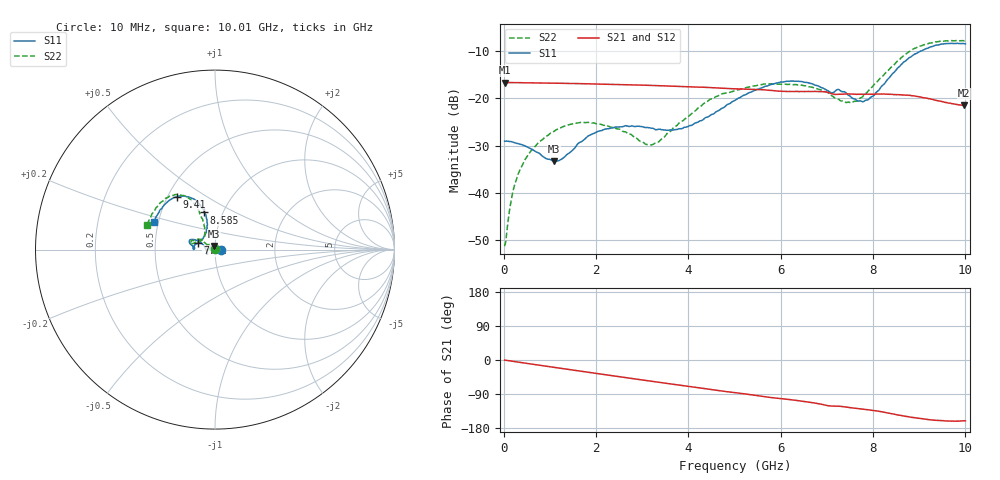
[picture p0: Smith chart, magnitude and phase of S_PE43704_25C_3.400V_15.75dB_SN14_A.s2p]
! Device ID: PE43704
! Dir: z:\PE43704\PE43704_Char_1_20130516\PE43704\AMB\3p400V\15p75dB
! Serial: 14
! Insertion: A
! Impedance: 50 ohm
! Temp: Amb
! VDD: 3.400V
! Attenuation Step: 15.75dB
! IDD: 1.139951e-01mA
#  Hz  S  RI  R  50
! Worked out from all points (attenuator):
!   401 points, 10 MHz to 10.01 GHz, reference 50 ohm
!   highest |S21| = -16.73 dB at 10 MHz (marker M1); lowest = -21.6 dB at 9.985 GHz (marker M2)
!   lowest |S11| = -33.3 dB at 1.085 GHz (marker M3), VSWR 1.04, Z = 49.4 + j2.07 ohm
!   |S11| at or under -10 dB: start of sweep to 9.074 GHz
!   |S22| runs from -51.2 to -7.9 dB; largest |S21 - S12| = 0.0013
!   S11 on the Smith chart (normalised r, x): 10 MHz: 1.07, +0.00; 7.51 GHz: 0.82, +0.06; 8.585 GHz: 0.82, +0.36; 9.41 GHz: 0.56, +0.38; 10.01 GHz: 0.47, +0.17
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1e7  0.0351 0.000273  0.1458 -0.000522  0.1459 -0.00048  -0.00269 0.000566
1.85e8  0.0336 0.00728  0.1452 -0.0087  0.1451 -0.00871  -0.00289 0.00969
3.6e8  0.0297 0.0133  0.1442 -0.0167  0.1441 -0.0169  -0.00614 0.0171
6.35e8  0.0192 0.0208  0.1416 -0.0288  0.1415 -0.0287  -0.0147 0.0258
1.085e9  -0.0054 0.0209  0.1353 -0.0477  0.1354 -0.0476  -0.0348 0.028
1.685e9  -0.0347 0.00293  0.1229 -0.0708  0.1229 -0.0706  -0.0543 0.0121
2.41e9  -0.045 -0.0203  0.1027 -0.0941  0.1027 -0.0941  -0.048 -0.00319
3.11e9  -0.0424 -0.0244  0.079 -0.1111  0.0791 -0.111  -0.0318 0.006
3.36e9  -0.0426 -0.0198  0.0697 -0.1156  0.0698 -0.1155  -0.0319 0.0139
4.035e9  -0.0513 0.00382  0.0443 -0.1235  0.0444 -0.1233  -0.0549 0.0369
4.46e9  -0.0614 0.0212  0.0282 -0.1261  0.0283 -0.1262  -0.0788 0.0555
5.01e9  -0.0848 0.0418  0.0083 -0.1246  0.0084 -0.1248  -0.1071 0.0529
5.96e9  -0.1344 0.0561  -0.023 -0.1161  -0.023 -0.1161  -0.134 0.0406
6.685e9  -0.138 0.0314  -0.0449 -0.1081  -0.0451 -0.1082  -0.1255 0.0334
7.51e9  -0.0973 0.0378  -0.0644 -0.0895  -0.0642 -0.0895  -0.0677 0.0584
7.86e9  -0.0626 0.0716  -0.0718 -0.0831  -0.0715 -0.0833  -0.0567 0.0974
8.36e9  -0.0446 0.1579  -0.0846 -0.0697  -0.0844 -0.07  -0.0763 0.1861
8.585e9  -0.0599 0.2071  -0.0894 -0.061  -0.0887 -0.0614  -0.101 0.234
8.935e9  -0.106 0.2733  -0.093 -0.0476  -0.093 -0.0468  -0.1626 0.2949
9.41e9  -0.2125 0.2925  -0.088 -0.0328  -0.0881 -0.0324  -0.2628 0.2905
9.985e9  -0.3336 0.1661  -0.0788 -0.0281  -0.0793 -0.0278  -0.3718 0.1445
1.001e10  -0.3396 0.1562  -0.0793 -0.0279  -0.0796 -0.0287  -0.3763 0.1359
